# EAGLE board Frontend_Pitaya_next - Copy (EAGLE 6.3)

Size 61.27 x 115.99 mm. Coordinates in mm from the lower left corner, seen from the top.
Outline: 0,0 61.27,0 61.27,110.32 arc42 0,110.32 0,0
Copper layers (1*16): Top 0.035mm / dielectric 1.5mm / Bottom 0.035mm
Design rules "default": minimum track width 10mil, minimum drill 24mil, track to track 8mil, track to pad 8mil, pad to pad 8mil, via to via 8mil, smd to smd 8mil, copper to edge 40mil, drill to drill 8mil, minimum pad ring 10mil, minimum via ring 8mil, stop-mask expansion 4mil, vias tented up to drill 0mil, thermal gap 10mil
Holes 3.2 mm at 2.54,97.8 57.15,97.8 2.54,13.8 57.15,13.8

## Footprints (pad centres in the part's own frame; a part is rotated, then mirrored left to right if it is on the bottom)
085CS_1AR = smd 2.9 x 2.5: + 3.25,0; - -3.25,0
C0805 = smd 1.3 x 1.5: 1 -0.85,0; 2 0.85,0
FE13-2 = drill 0.914: 1 -15.24,1.27 | drill 0.914 octagon: 2 -15.24,-1.27; 3 -12.7,1.27; 4 -12.7,-1.27; 5 -10.16,1.27; 6 -10.16,-1.27; 7 -7.62,1.27; 8 -7.62,-1.27; 9 -5.08,1.27; 10 -5.08,-1.27; 11 -2.54,1.27; 12 -2.54,-1.27; 13 0,1.27; 14 0,-1.27; 15 2.54,1.27; 16 2.54,-1.27; 17 5.08,1.27; 18 5.08,-1.27; 19 7.62,1.27; 20 7.62,-1.27; 21 10.16,1.27; 22 10.16,-1.27; 23 12.7,1.27; 24 12.7,-1.27; 25 15.24,1.27; 26 15.24,-1.27
D2PACK = smd 2.083 x 3.81: 1 -2.54,-8.89; 3 2.54,-8.89 | smd 11.43 x 8.89: 2 0,2.54
R0805 = smd 1.3 x 1.5: 1 -0.85,0; 2 0.85,0
MA03-1 = drill 1.016 long: 1 -2.54,0; 2 0,0; 3 2.54,0
JAE_NEXT = smd 2.54 x 0.406: 3V3 -2.748,1.155; 5VA -2.748,2.755; 5VB -2.748,1.955; A+ 2.337,-1.245; A- 2.337,-0.445; CV+ 2.337,-3.645; CV- 2.337,-2.845; G1 2.337,2.755; G3 2.337,1.955; G5 2.337,1.155; G7 2.337,0.355; G8 -2.748,0.355; G13 2.337,-2.045; G14 -2.748,-2.045; G19 2.337,-4.445; G20 -2.748,-4.445; SC+ -2.748,-3.645; SC- -2.748,-2.845; SD+ -2.748,-1.245; SD- -2.748,-0.445 | smd 2.54 x 2.54: P$1 -0.071,7.62; P$2 -0.071,-9.017 | hole 0.8: -0.205,3.455 | hole 1: -0.205,-5.045
MOLEX87833NEXT = drill 0.9: P$1 -1.27,1.27; P$2 -1.27,3.27; P$3 0.73,1.27; P$4 0.73,3.27; P$5 2.73,1.27; P$6 2.73,3.27; P$7 4.73,1.27; P$8 4.73,3.27
SN65LVDS105 = smd 1.524 x 0.635: P$1 -2.54,8.89; P$2 -2.54,7.62; P$3 -2.54,6.35; P$4 -2.54,5.08; P$5 -2.54,3.81; P$6 -2.54,2.54; P$7 -2.54,1.27; P$8 -2.54,0; P$9 3.81,0; P$10 3.81,1.27; P$11 3.81,2.54; P$12 3.81,3.81; P$13 3.81,5.08; P$14 3.81,6.35; P$15 3.81,7.62; P$16 3.81,8.89
EZG-00-302 = drill 0.6 pad 1: 1 0,-0.035; 2 -2.54,-2.505 | drill 0.9 pad 1.2: M1 -2.54,2.54; M2 2.54,2.54; M3 2.54,-2.54; M4 -2.54,-2.54

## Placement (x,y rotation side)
C1  100uF  [085CS_1AR]  29.21,36.83 0 bottom
C2  100nF  [C0805]  38.1,60.96 270 bottom
C3  100nF  [C0805]  33.02,43.18 0 bottom
C4  100nF  [C0805]  25.4,43.18 0 bottom
C5  100uF  [085CS_1AR]  29.21,26.67 180 bottom
E1  [FE13-2]  3.81,74.5 90 bottom
E2  [FE13-2]  55.88,74.5 90 bottom
E2_EXT  [FE13-2]  55.88,35.56 90 bottom
IC2  LD117AD2MTR  [D2PACK]  43.18,35.56 180 bottom
R1  150  [R0805]  36.83,49.53 0 bottom
R2  150  [R0805]  45.72,50.8 180 bottom
R3  150  [R0805]  36.83,55.88 0 bottom
R4  150  [R0805]  40.64,52.07 0 bottom
R5  100  [R0805]  45.72,55.88 0 bottom
R6  150  [R0805]  17.78,74.93 0 bottom
R7  150  [R0805]  12.7,74.93 0 bottom
SV1  [MA03-1]  38.1,3.81 270 top
SV2  [MA03-1]  22.86,3.81 270 top
SV3  [MA03-1]  8.89,3.81 270 top
SV4  [MA03-1]  5.08,52.07 0 top
SV5  [MA03-1]  5.08,43.18 0 top
SV6  [MA03-1]  5.08,35.56 0 top
SV7  [MA03-1]  5.08,26.67 0 top
U$1  JAE_NEXT  [JAE_NEXT]  13.97,92.46 0 top
U$2  MOLEX87833_NEXT  [MOLEX87833NEXT]  11.43,17.78 270 top
U$3  SN65LVDS105  [SN65LVDS105]  27.94,55.88 0 bottom
U$4  MOLEX87833_NEXT  [MOLEX87833NEXT]  25.4,17.78 270 top
U$5  JAE_NEXT  [JAE_NEXT]  27.94,92.46 0 top
U$6  MOLEX87833_NEXT  [MOLEX87833NEXT]  39.37,17.78 270 top
U$7  JAE_NEXT  [JAE_NEXT]  41.91,92.46 0 top
X1  EZG-00-302  [EZG-00-302]  44.45,3.81 0 top
X2  EZG-00-302  [EZG-00-302]  29.21,3.81 0 top
X3  EZG-00-302  [EZG-00-302]  15.24,3.81 0 top
X4  EZG-00-302  [EZG-00-302]  57.15,106.68 0 top
X5  EZG-00-302  [EZG-00-302]  49.53,106.68 0 top
X6  EZG-00-302  [EZG-00-302]  41.91,106.68 0 top
X7  EZG-00-302  [EZG-00-302]  34.29,106.68 0 top
X8  EZG-00-302  [EZG-00-302]  26.67,106.68 0 top
X9  EZG-00-302  [EZG-00-302]  19.05,106.68 0 top
X10  EZG-00-302  [EZG-00-302]  11.43,106.68 0 top
X11  EZG-00-302  [EZG-00-302]  3.81,106.68 0 top

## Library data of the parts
C1-C5 R1-R7 = resistor
E1 E2 E2_EXT = con-lsta; OC_FARNELL: unknown; OC_NEWARK: unknown
IC2 = v-reg
SV1-SV7 = con-lstb; OC_FARNELL: unknown; OC_NEWARK: unknown
U$1 U$5 U$7 = JAE_pad_extend
U$2 U$4 U$6 = molex 87833 next
U$3 = SN65LVDS105
X1-X11 = con-lemo; OC_FARNELL: unknown; OC_NEWARK: unknown

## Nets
3V3_A: IC2.2 SV7.3
3V3_B: E1.1 E1.2 SV7.1
+3V3: C1.+ C2.1 C4.1 R1.2 R3.2 SV7.2 U$1.3V3 U$3.P$1 U$3.P$2 U$3.P$3 U$3.P$4 U$3.P$8 U$5.3V3 U$7.3V3
+5V: C3.1 C5.+ E2.1 E2_EXT.1 IC2.3 U$1.5VA U$1.5VB U$5.5VA U$5.5VB U$7.5VA U$7.5VB
-4V: E2.2 E2_EXT.2
AN_IN_0: E2.13 X4.1
AN_IN_1: E2.14 X5.1
AN_IN_2: E2.15 X6.1
AN_IN_3: E2.16 X7.1
AN_OUT_0: E2.17 X8.1
AN_OUT_1: E2.18 X9.1
AN_OUT_2: E2.19 X10.1
AN_OUT_3: E2.20 X11.1
EXT_ADC_CLK+: E2.23 E2_EXT.23
EXT_ADC_CLK-: E2.24 E2_EXT.24
EXT_COM_MODE_GND: E2.11 E2_EXT.11
GND: C1.- C2.2 C3.2 C4.2 C5.- E1.25 E1.26 E2.12 E2.21 E2.22 E2.25 E2.26 E2_EXT.12 E2_EXT.21 E2_EXT.22 E2_EXT.25 E2_EXT.26 IC2.1 R2.1 R4.1 SV4.2 SV5.2 SV6.2 U$1.G1 U$1.G3 U$1.G5 U$1.G7 U$1.G8 U$1.G13 U$1.G14 U$1.G19 U$1.G20 U$3.P$5 U$5.G1 U$5.G3 U$5.G5 U$5.G7 U$5.G8 U$5.G13 U$5.G14 U$5.G19 U$5.G20 U$7.G1 U$7.G3 U$7.G5 U$7.G7 U$7.G8 U$7.G13 U$7.G14 U$7.G19 U$7.G20 X4.2 X5.2 X6.2 X7.2 X8.2 X9.2 X10.2 X11.2
GND_A1: SV1.2 U$6.P$1 U$6.P$2 U$6.P$3 U$6.P$5 U$6.P$7 U$6.P$8
GND_A2: SV2.2 U$4.P$1 U$4.P$2 U$4.P$3 U$4.P$5 U$4.P$7 U$4.P$8
GND_A3: SV3.2 U$2.P$1 U$2.P$2 U$2.P$3 U$2.P$5 U$2.P$7 U$2.P$8
I2C_SCL: E2_EXT.9
I2C_SDA: E2.10 E2_EXT.10
N$1: SV1.3 U$6.P$4 X1.2
N$9: E1.17 R6.2
N$11: E1.18 R7.2
N$24: SV1.1 U$6.P$6 X1.1
N$27: SV2.3 U$4.P$4 X2.2
N$30: SV4.1 U$3.P$16 U$7.CV+
N$31: SV4.3 U$3.P$15 U$7.CV-
N$32: SV2.1 U$4.P$6 X2.1
N$33: SV3.3 U$2.P$4 X3.2
N$34: R3.1 R4.2 R5.1 R7.1 U$3.P$7
N$35: SV5.1 U$3.P$14 U$5.CV+
N$36: SV3.1 U$2.P$6 X3.1
N$37: SV5.3 U$3.P$13 U$5.CV-
N$38: SV6.1 U$1.CV+ U$3.P$12
N$39: SV6.3 U$1.CV- U$3.P$11
N$40: R1.1 R2.2 R5.2 R6.1 U$3.P$6
RS_N: E1.14 U$1.A- U$5.A- U$7.A-
RS_P: E1.13 U$1.A+ U$5.A+ U$7.A+
SC_N_CH1: E1.8 U$7.SC-
SC_N_CH2: E1.6 U$5.SC-
SC_N_CH3: E1.10 U$1.SC-
SC_P_CH1: E1.7 U$7.SC+
SC_P_CH2: E1.5 U$5.SC+
SC_P_CH3: E1.9 U$1.SC+
SD_N_CH1: E1.4 U$7.SD-
SD_N_CH2: E1.12 U$5.SD-
SD_N_CH3: E1.16 U$1.SD-
SD_P_CH1: E1.3 U$7.SD+
SD_P_CH2: E1.11 U$5.SD+
SD_P_CH3: E1.15 U$1.SD+
SPI_CLK: E2.5 E2_EXT.5
SPI_CS: E2.6 E2_EXT.6
SPI_MIS0: E2.4 E2_EXT.4
SPI_MOSI: E2.3 E2_EXT.3
UART_RX: E2.8 E2_EXT.8
UART_TX: E2.7 E2.9 E2_EXT.7

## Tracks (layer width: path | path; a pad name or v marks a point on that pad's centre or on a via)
3V3_A  (1 unrouted)
3V3_B  (2 unrouted)
+3V3  (13 unrouted)
+5V  (10 unrouted)
-4V  (1 unrouted)
AN_IN_0  (1 unrouted)
AN_IN_1  (1 unrouted)
AN_IN_2  (1 unrouted)
AN_IN_3  (1 unrouted)
AN_OUT_0  (1 unrouted)
AN_OUT_1  (1 unrouted)
AN_OUT_2  (1 unrouted)
AN_OUT_3  (1 unrouted)
EXT_ADC_CLK+  (1 unrouted)
EXT_ADC_CLK-  (1 unrouted)
EXT_COM_MODE_GND  (1 unrouted)
GND  (58 unrouted)
GND_A1  (6 unrouted)
GND_A2  (6 unrouted)
GND_A3  (6 unrouted)
I2C_SDA  (1 unrouted)
N$1  (2 unrouted)
N$9  (1 unrouted)
N$11  (1 unrouted)
N$24  (2 unrouted)
N$27  (2 unrouted)
N$30  (2 unrouted)
N$31  (2 unrouted)
N$32  (2 unrouted)
N$33  (2 unrouted)
N$34  (4 unrouted)
N$35  (2 unrouted)
N$36  (2 unrouted)
N$37  (2 unrouted)
N$38  (2 unrouted)
N$39  (2 unrouted)
N$40  (4 unrouted)
RS_N  (3 unrouted)
RS_P  (3 unrouted)
SC_N_CH1  (1 unrouted)
SC_N_CH2  (1 unrouted)
SC_N_CH3  (1 unrouted)
SC_P_CH1  (1 unrouted)
SC_P_CH2  (1 unrouted)
SC_P_CH3  (1 unrouted)
SD_N_CH1  (1 unrouted)
SD_N_CH2  (1 unrouted)
SD_N_CH3  (1 unrouted)
SD_P_CH1  (1 unrouted)
SD_P_CH2  (1 unrouted)
SD_P_CH3  (1 unrouted)
SPI_CLK  (1 unrouted)
SPI_CS  (1 unrouted)
SPI_MIS0  (1 unrouted)
SPI_MOSI  (1 unrouted)
UART_RX  (1 unrouted)
UART_TX  (2 unrouted)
